(* Logix 5000 Rung export; software revision 16.03 *)

MODULES
   RemoteENBT : vendor None type None code None
   MNETR : vendor None type None code None
END_MODULES

TYPE MNETRIPADDRESS :   // Data structure to get and set the IP address of the module.
STRUCT
   IPGetTrigger : BOOL;   // Gets IP address.
   IPReceived : INT[4];   // IP address received.
   IPSetTrigger : BOOL;   // Sets IP address
   IPRequested : INT[4];   // IP address set.
END_STRUCT
END_TYPE

TYPE MNETRDATA :   // Contains Read Data (data read from the module to the processor) and Write Data (data written from the processor to the module)
STRUCT
   ReadData : INT[600];   // Data read from module
   WriteData : INT[600];   // Data to write to module
END_STRUCT
END_TYPE

TYPE MNETRCMDCONTROL :   // Controlling the Modbus Commands
STRUCT
   CmdIndex : INT[6];   // Stores the command indexes for command control.
   NumberOfCommands : INT;   // Number of commands per block (1 to 6)
   CommandsAddedtoQueue : INT;   // Number of commands added to queue
   CmdControlTrigger : BOOL;   // Trigger Command Control. User application will activate this trigger.
END_STRUCT
END_TYPE

TYPE MNETRBLOCKSTATS :   // This object is used to store the block transfer statistics for the MVI56-MNETR module.
STRUCT
   Read : INT;   // Total number of read block transfers
   Write : INT;   // Total number of write block transfers
   Parse : INT;   // Total number of blocks parsed
   Event : INT;   // Total number of event blocks received
   Cmd : INT;   // Total number of command blocks received
   Err : INT;   // Total number of block transfer errors
END_STRUCT
END_TYPE

TYPE MNETRSTATUS :   // This status data is returned on each read block and can be used to detect proper module operation.
STRUCT
   PassCnt : INT;   // Program cycle counter
   ProductVersion : INT;   // Shows the module software version
   ProductCode : INT[2];   // This identifies the module product code
   BlockStats : MNETRBLOCKSTATS;   // Block Transfer Statistics.
   Reserved1 : INT;   // Reserved INT
   Reserved2 : INT;   // Reserved INT
   MNetReq : INT;   // number of remote client requests for port 502
   MNetResp : INT;   // number of server responses for port 502
   MBAPReq : INT;   // number of remote client requests for port 2000
   MBAPResp : INT;   // number of server responses for port 2000
   ClientStatus : MNETRCLIENTSTATS;   // Client Status
END_STRUCT
END_TYPE

TYPE MNETRMODULEDEF :   // this defines the whole module which includes all tags used in the program
STRUCT
   DATA : MNETRDATA;   // Data read from module
   STATUS : MNETRSTATUS;   // Client ,Server Status and blocks status
   CONTROL : MNETRCONTROL;   // Module control warmboot, coldboot, etc
   UTIL : MNETRUTIL;   // command, event control
END_STRUCT
END_TYPE

TYPE MNETRUTIL :   // Variables for internal ladder usage - should not be accessed by user application
STRUCT
   LastRead : INT;   // Index of last read block
   LastWrite : INT;   // Index of last write block
   BlockIndex : INT;   // Computed block offset for data table
   ReadDataSizeGet : INT;   // Gets ReadData Array Length.
   WriteDataSizeGet : INT;   // Gets WriteData Array Length.
   ReadDataBlkCount : INT;   // Holds the value of the Block Counts of the Read Data Array. Array Size is divided by 40.
   WriteDataBlkCount : INT;   // Holds the value of the Block Counts of the Write Data Array. Array Size is divided by 40.
   RBTSremainder : INT;   // Holds remainder calculation value from the read array.
   WBTSremainder : INT;   // Holds remainder calculation value from the write array.
   IPsetPending : BOOL;   // Allows Setting module IP address
   IPgetPending : BOOL;   // Allows Getting module IP address
   InitOutBlkIDLim : INT;   // Block Index Limit for ReadData size of the array
END_STRUCT
END_TYPE

TYPE MNETRCOILARRAY :   // Conversion to INT values
STRUCT
   Boolean : BOOL[416];   // Conversion from Bool to INT data types
END_STRUCT
END_TYPE

TYPE MNETRCLIENTSTATS :   // This object is used to store client statistics for the MVI56-MNETR module.
STRUCT
   CmdReq : INT;   // Total number of command list requests sent
   CmdResp : INT;   // Total number of command list responses received
   CmdErr : INT;   // Total number of command list errors
   Requests : INT;   // Total number of requests for port
   Responses : INT;   // Total number of responses for port
   ErrSent : INT;   // Total number of errors sent
   ErrRec : INT;   // Total number of errors received
   CfgErrWord : INT;   // Configuration Error Word
   CurErr : INT;   // Current Error code
   LastErr : INT;   // Last recorded error code
END_STRUCT
END_TYPE

TYPE MNETREVENTCMD :   // Data structure to use for Event message generation.
STRUCT
   IP0 : INT;   // First digit of IP address
   IP1 : INT;   // Second digit of IP address
   IP2 : INT;   // Third digit of IP address
   IP3 : INT;   // Last digit of IP address
   ServPort : INT;   // TCP Service Port number (0-65535), 502 for MBAP, 2000 for MNET
   Node : INT;   // Modbus slave node address (0 to 247)
   DBAddress : INT;   // Module internal database to use with message
   Count : INT;   // Register or data point count
   Swap : INT;   // Swap code to use with functions 3 and 4
   Function : INT;   // Modbus function code for message
   Address : INT;   // Address to interface with in device
   Result : INT;   // shows the result of the event that was sent
END_STRUCT
END_TYPE

TYPE MNETRPASSTHRU :   // Applicable with the selection of a Pass-Through mode (1 to 3) in the Configuration file.
STRUCT
   MBControl1 : CONTROL;   // Modbus pass thru message control
   MBControl2 : CONTROL;   // Modbus pass thru message control
   MBMsg : SINT[500];   // message array
   MBScratch : INT[3];   // temporary used ints
   MBOffsetBit : INT;   // offset bit in the message
   MBOffset : INT;   // start offset in the message
   MBMsgLen : INT;   // message length
   mbdouble : DINT;   // Modbus double int tag
   MBCoil : MNETRCOILARRAY;   // Conversion array
END_STRUCT
END_TYPE

TYPE MNETRCONTROL :   // Module Behaviour Control Tags. Values used by program for data transfer operation between the module and the processor.
STRUCT
   BootTimer : TIMER;   // Starts counting when user issues a coldboot or warmboot
   WarmBoot : BOOL;   // Causes software reset. The Module reads new configuration information.
   ColdBoot : BOOL;   // Causes hardware reset.
   EventCmdTrigger : BOOL;   // Trigger events to be executed by the module
   EventCmd : MNETREVENTCMD;   // Event command Data
   CmdControl : MNETRCMDCONTROL;   // Command control data
   PassThru : MNETRPASSTHRU;   // Pass thru data format
   IPAddress : MNETRIPADDRESS;   // Getting and Setting IP address to and from Module
END_STRUCT
END_TYPE

ADD_ON_INSTRUCTION AOI56MNETR   (* revision 1.3, vendor ProSoft Technology Inc., ExecutePrescan *)
// Add-On - MVI56-MNETR & MVI56E-MNETR modules
// Revision note:
// v1.3 - 1) flexible read and write data arrays, 2) Includes blocks 9990/9991
VAR_IN_OUT
   Connection_Input : INT[42]; {required}   // Input parameters.
   Connection_Output : INT[42]; {required}   // Output parameters.
   MNETR : MNETRMODULEDEF; {required}
END_VAR
VAR
   MJFAULTS : DINT[12];
END_VAR

ROUTINE Logic   (* ladder *)
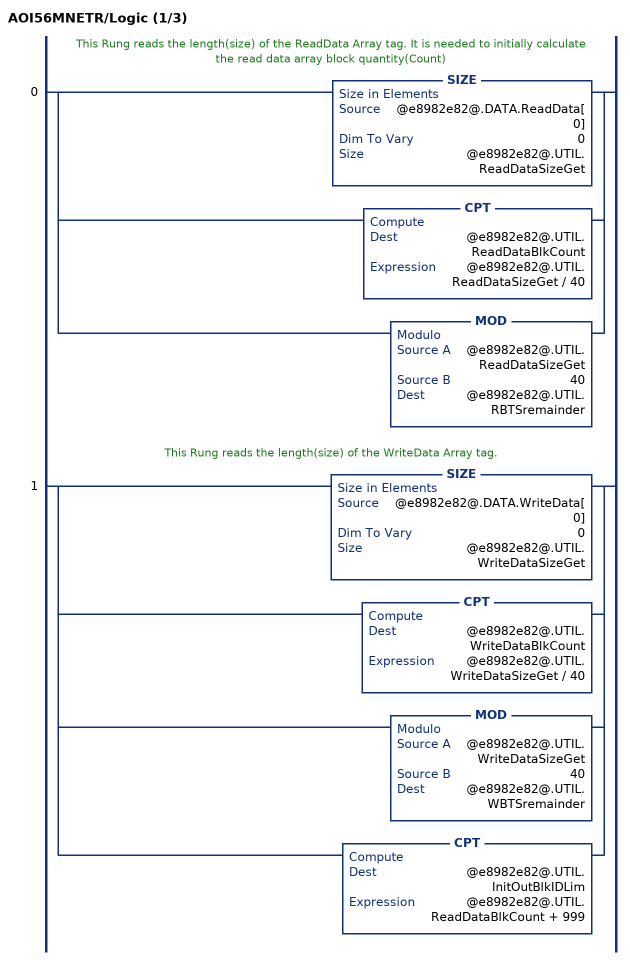
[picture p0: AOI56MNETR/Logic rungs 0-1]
   // This Rung reads the length(size) of the ReadData Array tag. It is needed to initially calculate the read data array block quantity(Count)
   0: [SIZE(@e8982e82@.DATA.ReadData[0],0,@e8982e82@.UTIL.ReadDataSizeGet) ,CPT(@e8982e82@.UTIL.ReadDataBlkCount,@e8982e82@.UTIL.ReadDataSizeGet / 40) ,MOD(@e8982e82@.UTIL.ReadDataSizeGet,40,@e8982e82@.UTIL.RBTSremainder) ];
   // This Rung reads the length(size) of the WriteData Array tag.
   1: [SIZE(@e8982e82@.DATA.WriteData[0],0,@e8982e82@.UTIL.WriteDataSizeGet) ,CPT(@e8982e82@.UTIL.WriteDataBlkCount,@e8982e82@.UTIL.WriteDataSizeGet / 40) ,MOD(@e8982e82@.UTIL.WriteDataSizeGet,40,@e8982e82@.UTIL.WBTSremainder) ,CPT(@e8982e82@.UTIL.InitOutBlkIDLim,@e8982e82@.UTIL.ReadDataBlkCount + 999) ];
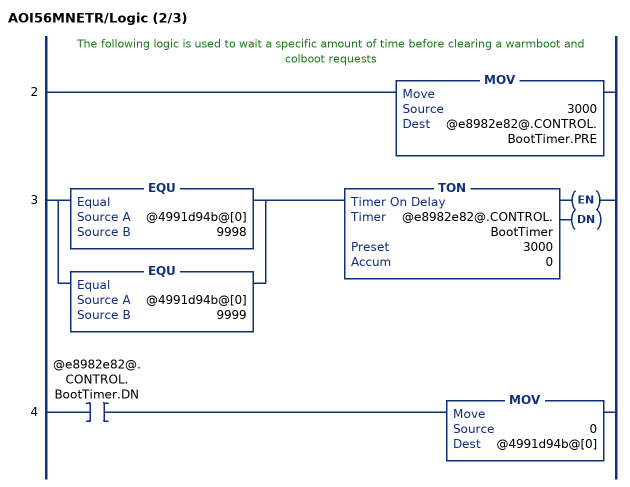
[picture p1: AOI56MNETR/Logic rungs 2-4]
   // The following logic is used to wait a specific amount of time before clearing a warmboot and colboot requests
   2: MOV(3000,@e8982e82@.CONTROL.BootTimer.PRE);
   3: [EQU(@4991d94b@[0],9998) ,EQU(@4991d94b@[0],9999) ]TON(@e8982e82@.CONTROL.BootTimer,3000,0);
   4: XIC(@e8982e82@.CONTROL.BootTimer.DN)MOV(0,@4991d94b@[0]);
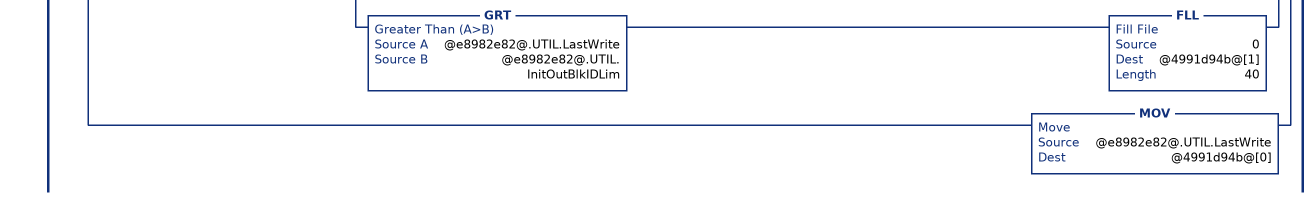
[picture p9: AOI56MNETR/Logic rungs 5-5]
   // This rung is used to check for a new read block from the MVI56-MNETR.  If new data is available, the LastRead and Input Image Word[41] will not be equal.  This will force the program to call the ReadData subroutine to process the new data received.  After the new data is placed in the ReadData controller tags, the program will send new data to the module using the WriteData subroutine.
   5: NEQ(@e611f268@[41],@e8982e82@.UTIL.LastRead)[MOV(@e611f268@[41],@e8982e82@.UTIL.LastRead) ,[EQU(-1,@e8982e82@.UTIL.LastRead) ,EQU(0,@e8982e82@.UTIL.LastRead) ] [COP(@e611f268@[1],@e8982e82@.STATUS.PassCnt,1) ,COP(@e611f268@[2],@e8982e82@.STATUS.BlockStats.Read,6) ,COP(@e611f268@[8],@e8982e82@.STATUS.Reserved1,6) ,COP(@e611f268@[14],@e8982e82@.STATUS.ClientStatus.CmdReq,10) ,COP(@e611f268@[24],@e8982e82@.STATUS.ProductCode[0],2) ,COP(@e611f268@[26],@e8982e82@.STATUS.ProductVersion,1) ] ,GEQ(@e8982e82@.UTIL.LastRead,1) [LEQ(@e8982e82@.UTIL.LastRead,@e8982e82@.UTIL.ReadDataBlkCount) [CPT(@e8982e82@.UTIL.BlockIndex,(@e8982e82@.UTIL.LastRead - 1) * 40) ,COP(@e611f268@[1],@e8982e82@.DATA.ReadData[@e8982e82@.UTIL.BlockIndex],40) ] ,CMP(@e8982e82@.UTIL.LastRead - @e8982e82@.UTIL.ReadDataBlkCount = 1) GRT(@e8982e82@.UTIL.RBTSremainder,0) [CPT(@e8982e82@.UTIL.BlockIndex,(@e8982e82@.UTIL.LastRead-1) * 40) ,COP(@e611f268@[1],@e8982e82@.DATA.ReadData[@e8982e82@.UTIL.BlockIndex],@e8982e82@.UTIL.RBTSremainder) ] ] ,EQU(@e8982e82@.UTIL.LastRead,9990) [COP(@e611f268@[1],@e8982e82@.CONTROL.IPAddress.IPRequested[0],4) ,OTU(@e8982e82@.UTIL.IPsetPending) ] ,EQU(@e8982e82@.UTIL.LastRead,9991) [COP(@e611f268@[1],@e8982e82@.CONTROL.IPAddress.IPReceived[0],4) ,OTU(@e8982e82@.UTIL.IPgetPending) ] ,EQU(@e8982e82@.UTIL.LastRead,2000) MOV(@e611f268@[1],@e8982e82@.CONTROL.EventCmd.Result) ,LIM(5001,@e8982e82@.UTIL.LastRead,5006) MOV(@e611f268@[1],@e8982e82@.CONTROL.CmdControl.CommandsAddedtoQueue) ,EQU(9996,@e8982e82@.UTIL.LastRead) [MOV(@e611f268@[1],@e8982e82@.CONTROL.PassThru.MBMsgLen) ,COP(@e611f268@[3],@e8982e82@.CONTROL.PassThru.MBMsg[0],@e8982e82@.CONTROL.PassThru.MBMsgLen) ] ,LIM(9956,@e8982e82@.UTIL.LastRead,9957) [MOV(@e611f268@[2],@e8982e82@.CONTROL.PassThru.MBOffset) ,LES(@e8982e82@.CONTROL.PassThru.MBOffset,@e8982e82@.UTIL.WriteDataSizeGet) COP(@e611f268@[3],@e8982e82@.DATA.WriteData[@e8982e82@.CONTROL.PassThru.MBOffset],@e611f268@[1]) ] ,EQU(9958,@e8982e82@.UTIL.LastRead) [MOV(@e611f268@[2],@e8982e82@.CONTROL.PassThru.MBOffsetBit) ,MOV(@e611f268@[3],@e8982e82@.CONTROL.PassThru.MBScratch[2]) ,DIV(@e8982e82@.CONTROL.PassThru.MBOffsetBit,16,@e8982e82@.CONTROL.PassThru.MBOffset) ,MOD(@e8982e82@.CONTROL.PassThru.MBOffsetBit,16,@e8982e82@.CONTROL.PassThru.MBOffsetBit) ,XPY(2,@e8982e82@.CONTROL.PassThru.MBOffsetBit,@e8982e82@.CONTROL.PassThru.mbdouble) ,MVM(@e8982e82@.CONTROL.PassThru.mbdouble,16#0000_ffff,@e8982e82@.CONTROL.PassThru.MBOffsetBit) ,NEQ(@e8982e82@.CONTROL.PassThru.MBScratch[2],0) OR(@e8982e82@.CONTROL.PassThru.MBOffsetBit,@e8982e82@.DATA.WriteData[@e8982e82@.CONTROL.PassThru.MBOffset],@e8982e82@.DATA.WriteData[@e8982e82@.CONTROL.PassThru.MBOffset]) ,EQU(@e8982e82@.CONTROL.PassThru.MBScratch[2],0) [NOT(@e8982e82@.CONTROL.PassThru.MBOffsetBit,@e8982e82@.CONTROL.PassThru.MBOffsetBit) ,AND(@e8982e82@.CONTROL.PassThru.MBOffsetBit,@e8982e82@.DATA.WriteData[@e8982e82@.CONTROL.PassThru.MBOffset],@e8982e82@.DATA.WriteData[@e8982e82@.CONTROL.PassThru.MBOffset]) ] ] ,EQU(9959,@e8982e82@.UTIL.LastRead) [MOV(@e611f268@[2],@e8982e82@.CONTROL.PassThru.MBOffset) ,MOV(@e611f268@[1],@e8982e82@.CONTROL.PassThru.MBControl1.LEN) ,MOV(@e611f268@[1],@e8982e82@.CONTROL.PassThru.MBControl2.LEN) ,FAL(@e8982e82@.CONTROL.PassThru.MBControl1,2,0,ALL,@e8982e82@.DATA.WriteData[@e8982e82@.CONTROL.PassThru.MBOffset+@e8982e82@.CONTROL.PassThru.MBControl1.POS],@e8982e82@.DATA.WriteData[@e8982e82@.CONTROL.PassThru.MBOffset+@e8982e82@.CONTROL.PassThru.MBControl1.POS] AND(NOT @e611f268@[14+@e8982e82@.CONTROL.PassThru.MBControl1.POS])) ,FAL(@e8982e82@.CONTROL.PassThru.MBControl2,2,0,ALL,@e8982e82@.DATA.WriteData[@e8982e82@.CONTROL.PassThru.MBOffset+@e8982e82@.CONTROL.PassThru.MBControl2.POS],@e8982e82@.DATA.WriteData[@e8982e82@.CONTROL.PassThru.MBOffset+@e8982e82@.CONTROL.PassThru.MBControl2.POS] OR(@e611f268@[14+@e8982e82@.CONTROL.PassThru.MBControl2.POS] AND @e611f268@[3+@e8982e82@.CONTROL.PassThru.MBControl2.POS])) ] ,EQU(9961,@e8982e82@.UTIL.LastRead) [MOV(@e611f268@[1],@e8982e82@.CONTROL.PassThru.MBMsgLen) ,CPT(@e8982e82@.CONTROL.PassThru.MBMsgLen,@e8982e82@.CONTROL.PassThru.MBMsgLen*2+2) ,COP(@e611f268@[3],@e8982e82@.CONTROL.PassThru.MBMsg[0],@e8982e82@.CONTROL.PassThru.MBMsgLen) ] ,MOV(@e611f268@[0],@e8982e82@.UTIL.LastWrite) ,XIC(@e8982e82@.CONTROL.WarmBoot) [MOV(9998,@e8982e82@.UTIL.LastWrite) ,OTU(@e8982e82@.CONTROL.WarmBoot) ] ,XIC(@e8982e82@.CONTROL.ColdBoot) [MOV(9999,@e8982e82@.UTIL.LastWrite) ,OTU(@e8982e82@.CONTROL.ColdBoot) ] ,XIC(@e8982e82@.CONTROL.IPAddress.IPSetTrigger) XIO(@e8982e82@.UTIL.IPsetPending) [COP(@e8982e82@.CONTROL.IPAddress.IPRequested[0],@4991d94b@[1],4) ,MOV(9990,@e8982e82@.UTIL.LastWrite) ,OTU(@e8982e82@.CONTROL.IPAddress.IPSetTrigger) ,OTL(@e8982e82@.UTIL.IPsetPending) ] ,XIC(@e8982e82@.CONTROL.IPAddress.IPGetTrigger) XIO(@e8982e82@.UTIL.IPgetPending) [MOV(9991,@e8982e82@.UTIL.LastWrite) ,OTU(@e8982e82@.CONTROL.IPAddress.IPGetTrigger) ,OTL(@e8982e82@.UTIL.IPgetPending) ] ,XIC(@e8982e82@.CONTROL.CmdControl.CmdControlTrigger) [CPT(@e8982e82@.UTIL.LastWrite,5000+@e8982e82@.CONTROL.CmdControl.NumberOfCommands) ,COP(@e8982e82@.CONTROL.CmdControl.CmdIndex[0],@4991d94b@[1],6) ,CPT(@4991d94b@[0],5000+@e8982e82@.CONTROL.CmdControl.NumberOfCommands) ,OTU(@e8982e82@.CONTROL.CmdControl.CmdControlTrigger) ] ,XIC(@e8982e82@.CONTROL.EventCmdTrigger) [MOV(2000,@e8982e82@.UTIL.LastWrite) ,COP(@e8982e82@.CONTROL.EventCmd.IP0,@4991d94b@[1],11) ,OTU(@e8982e82@.CONTROL.EventCmdTrigger) ] ,GEQ(@e8982e82@.UTIL.LastWrite,1) [LEQ(@e8982e82@.UTIL.LastWrite,@e8982e82@.UTIL.WriteDataBlkCount) [CPT(@e8982e82@.UTIL.BlockIndex,(@e8982e82@.UTIL.LastWrite - 1) * 40) ,COP(@e8982e82@.DATA.WriteData[@e8982e82@.UTIL.BlockIndex],@4991d94b@[1],40) ] ,CMP(@e8982e82@.UTIL.LastWrite - @e8982e82@.UTIL.WriteDataBlkCount = 1) GRT(@e8982e82@.UTIL.WBTSremainder,0) [CPT(@e8982e82@.UTIL.BlockIndex,(@e8982e82@.UTIL.LastWrite-1) * 40) ,COP(@e8982e82@.DATA.WriteData[@e8982e82@.UTIL.BlockIndex],@4991d94b@[1],@e8982e82@.UTIL.WBTSremainder) ] ] ,LIM(1000,@e8982e82@.UTIL.LastWrite,1124) [LEQ(@e8982e82@.UTIL.LastWrite,@e8982e82@.UTIL.InitOutBlkIDLim) [CPT(@e8982e82@.UTIL.BlockIndex,(@e8982e82@.UTIL.LastWrite - 1000) * 40) ,COP(@e8982e82@.DATA.ReadData[@e8982e82@.UTIL.BlockIndex],@4991d94b@[1],40) ] ,GRT(@e8982e82@.UTIL.LastWrite,@e8982e82@.UTIL.InitOutBlkIDLim) FLL(0,@4991d94b@[1],40) ] ,MOV(@e8982e82@.UTIL.LastWrite,@4991d94b@[0]) ];
END_ROUTINE

ROUTINE Prescan   (* ladder *)
// Prescan
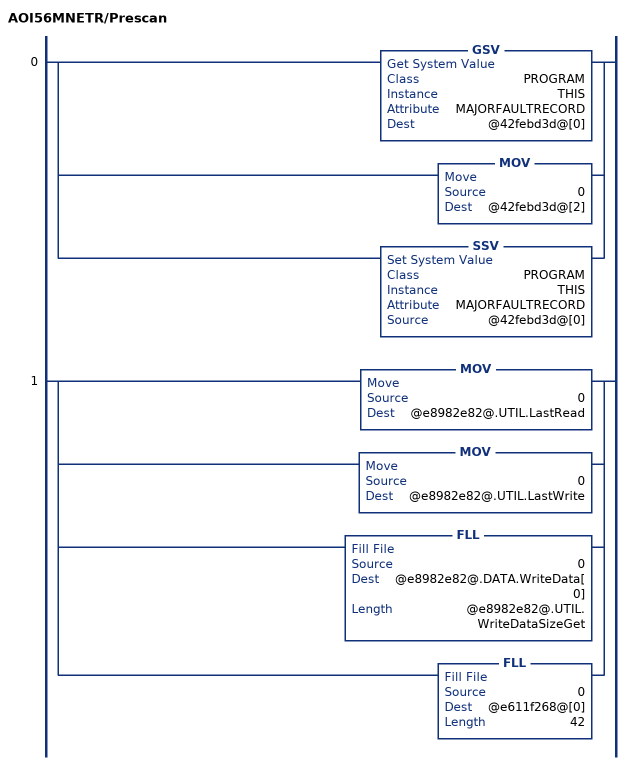
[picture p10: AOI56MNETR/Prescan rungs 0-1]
   0: [GSV(PROGRAM,THIS,MAJORFAULTRECORD,@42febd3d@[0]) ,MOV(0,@42febd3d@[2]) ,SSV(PROGRAM,THIS,MAJORFAULTRECORD,@42febd3d@[0]) ];
   1: [MOV(0,@e8982e82@.UTIL.LastRead) ,MOV(0,@e8982e82@.UTIL.LastWrite) ,FLL(0,@e8982e82@.DATA.WriteData[0],@e8982e82@.UTIL.WriteDataSizeGet) ,FLL(0,@e611f268@[0],42) ];
END_ROUTINE
END_ADD_ON_INSTRUCTION

VAR_GLOBAL   (* controller tags *)
   RemoteENBT:1:I : AB:1756_MODULE_INT_84Bytes:I:0;
   MNETR : MNETRMODULEDEF;
   RemoteENBT:1:O : AB:1756_MODULE_INT_84Bytes:O:0;
   AOI56MNETR : AOI56MNETR;
END_VAR

PROGRAM MainProgram

ROUTINE MainRoutine   (* ladder *)
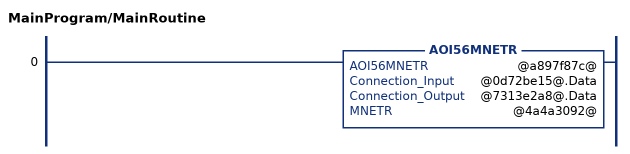
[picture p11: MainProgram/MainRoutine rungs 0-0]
   0: AOI56MNETR(@a897f87c@,@0d72be15@.Data,@7313e2a8@.Data,@4a4a3092@);
END_ROUTINE
END_PROGRAM
